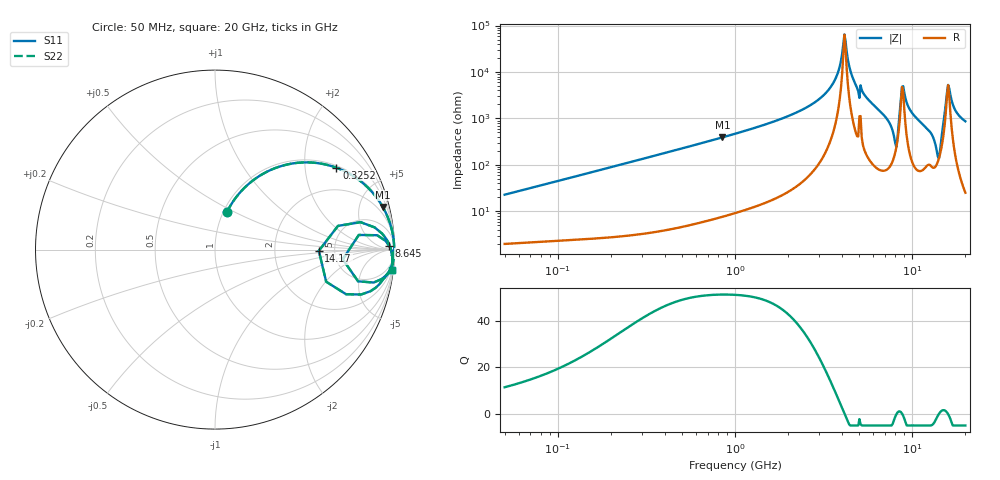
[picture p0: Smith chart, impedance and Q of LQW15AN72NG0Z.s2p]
!Murata Part Number: LQW15AN72NG0Z
!These Parameters are Measured in Series Mode Connection
!  o--[Z]--o
!Port1  Port2
!  o-------o
!Freq. Start=50[MHz] Stop=20[GHz], 401[Steps]
# Hz S RI R 50
!Freq.(Hz) S11(Real) S11(Imag) S21(Real) S21(Imag) S12(Real) S12(Imag) S22(Real) S22(Imag)
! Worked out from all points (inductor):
!   401 points, 50 MHz to 20 GHz, reference 50 ohm
!   read as one part in series: L = 72 nH near 51.52 MHz
!   highest Q = 51.4 at 848.1 MHz (marker M1), where L = 73.3 nH
!   self-resonance near 4.149 GHz
!   S11 on the Smith chart (normalised r, x): 50 MHz: 1.04, +0.45; 325.2 MHz: 1.07, +2.91; 8.645 GHz: 42, +32; 14.17 GHz: 3.74, -0.07; 20 GHz: 2, -17
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5e7  0.0658 0.208  0.9342 -0.208  0.9342 -0.208  0.0658 0.208
1.364002e8  0.2805 0.4294  0.7195 -0.4294  0.7195 -0.4294  0.2805 0.4294
3.251725e8  0.6762 0.4564  0.3238 -0.4564  0.3238 -0.4564  0.6762 0.4564
3.721004e8  0.7315 0.4322  0.2685 -0.4322  0.2685 -0.4322  0.7315 0.4322
8.480927e8  0.9345 0.2379  0.0655 -0.2379  0.0655 -0.2379  0.9345 0.2379
1e9  0.9526 0.2029  0.0474 -0.2029  0.0474 -0.2029  0.9526 0.2029
2.728004e9  0.996 0.0487  0.00403 -0.0487  0.00403 -0.0487  0.996 0.0487
3.626126e9  0.9982 0.0159  0.00176 -0.0159  0.00176 -0.0159  0.9982 0.0159
3.850025e9  0.9984 0.00901  0.00159 -0.00901  0.00159 -0.00901  0.9984 0.00901
4.149438e9  0.9985 0.000236  0.00153 -0.000236  0.00153 -0.000236  0.9985 0.000236
4.89267e9  0.9975 -0.0219  0.0025 0.0219  0.0025 0.0219  0.9975 -0.0219
7.442007e9  0.9722 -0.1181  0.0278 0.1181  0.0278 0.1181  0.9722 -0.1181
8.141811e9  0.7118 -0.0537  0.2882 0.0537  0.2882 0.0537  0.7118 -0.0537
8.644534e9  0.9701 0.0224  0.0299 -0.0224  0.0299 -0.0224  0.9701 0.0224
9.041845e9  0.9874 -0.0248  0.0126 0.0248  0.0126 0.0248  0.9874 -0.0248
9.892087e9  0.9883 -0.0702  0.0117 0.0702  0.0117 0.0702  0.9883 -0.0702
1.334722e10  0.8658 -0.232  0.1342 0.232  0.1342 0.232  0.8658 -0.232
1.417136e10  0.5785 -0.00665  0.4215 0.00665  0.4215 0.00665  0.5785 -0.00665
1.482269e10  0.8894 0.1237  0.1106 -0.1237  0.1106 -0.1237  0.8894 0.1237
1.597544e10  0.9815 -0.00224  0.0185 0.00224  0.0185 0.00224  0.9815 -0.00224
1.774144e10  0.9886 -0.0701  0.0114 0.0701  0.0114 0.0701  0.9886 -0.0701
2e10  0.9837 -0.1129  0.0163 0.1129  0.0163 0.1129  0.9837 -0.1129
